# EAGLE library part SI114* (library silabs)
PROXIMITY/UV/AMBIENT LIGHT SENSOR IC WITH I2C INTERFACE Source: http://www.silabs.com/Support%20Documents/TechnicalDocs/Si1145-46-47.pdf
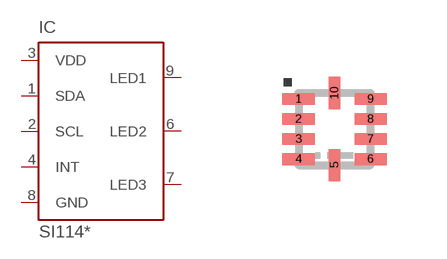
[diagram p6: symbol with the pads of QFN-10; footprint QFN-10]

Designator prefix IC

## SI1145, SI1146, SI1147  [QFN-10]
1  SDA
2  SCL  in
3  VDD  pwr
4  INT  oc
6  LED2  out
7  LED3  out
8  GND  pwr
9  LED1  out

## Footprint QFN-10 (pad centres in mm)
10-Pin QFN Source: http://www.silabs.com/Support%20Documents/TechnicalDocs/Si1145-46-47.pdf
smd 0.8 x 0.3: 1 -0.9,0.75; 2 -0.9,0.25; 3 -0.9,-0.25; 4 -0.9,-0.75; 6 0.9,-0.75; 7 0.9,-0.25; 8 0.9,0.25; 9 0.9,0.75
smd 0.3 x 0.8: 5 0,-0.9; 10 0,0.9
